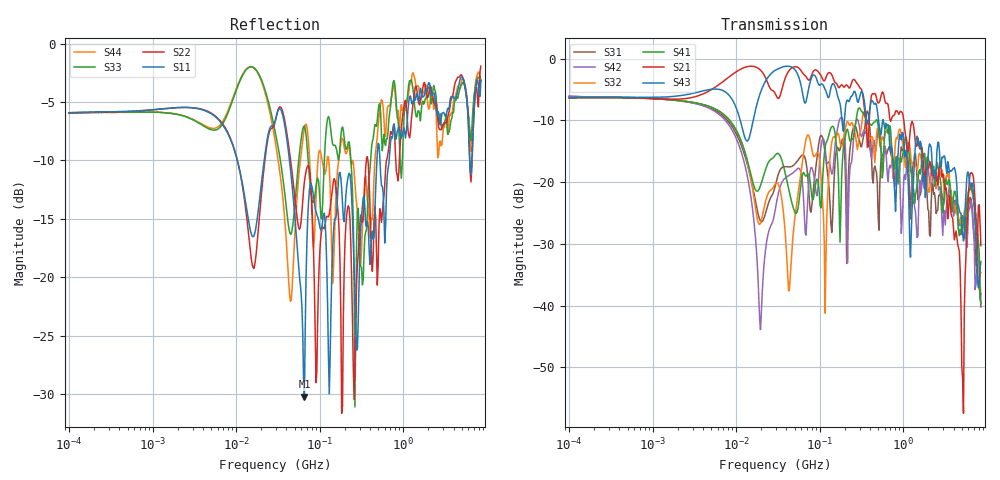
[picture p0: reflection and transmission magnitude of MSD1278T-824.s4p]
# MHz S MA R 50
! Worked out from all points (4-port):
!   498 points, 100 kHz to 8.5 GHz, reference 50 ohm
!   strongest paths, dB at 100 kHz, 1.698 MHz, 29.49 MHz, 500.7 MHz, 8.5 GHz:
!     S43: -6.3, -6.2, -1.9, -9.5, -32.8
!     S21: -6.4, -6.6, -5.7, -7.2, -30.3
!     S41: -6.4, -6.7, -15.6, -10.9, -39.5
!     S32: -6.4, -6.7, -20.3, -11.3, -34.7
!     S42: -6.1, -6.7, -24.4, -11.4, -38.0
!     S31: -6.1, -6.7, -20.5, -25.5, -40.2
!   lowest |S11| = -30.2 dB at 65.59 MHz (marker M1), VSWR 1.06, Z = 53.1 + j0.452 ohm
!   |S11| at or under -10 dB: 43.46 MHz to 484.3 MHz (440.9 MHz wide, 167 % of centre); 526.4 MHz to 678.1 MHz (151.7 MHz wide, 25.2 % of centre); 6.252 GHz to 6.618 GHz (365.6 MHz wide, 5.68 % of centre)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
0.1  0.5059 5.4  0.4812 6.1  0.4951 -7.2  0.4807 -175.5
     0.4812 6.1  0.5047 5.5  0.4805 -175.5  0.4953 -7.3
     0.4951 -7.2  0.4805 -175.5  0.5051 5.5  0.4826 6.0
     0.4807 -175.5  0.4953 -7.3  0.4826 6.0  0.5036 5.6
19.54962  0.2337 17.6  0.8058 -13.1  0.04836 -163.0  0.09366 69.0
          0.8058 -13.1  0.2051 29.1  0.04652 57.7  0.006398 29.0
          0.04836 -163.0  0.04652 57.7  0.7153 -33.3  0.5315 38.2
          0.09366 69.0  0.006398 29.0  0.5315 38.2  0.7061 -40.8
42.49738  0.3387 -68.9  0.7908 6.8  0.1325 92.8  0.08804 2.7
          0.7908 6.8  0.3657 -54.3  0.01314 43.2  0.1123 98.1
          0.1325 92.8  0.01314 43.2  0.1639 -37.2  0.8664 -8.5
          0.08804 2.7  0.1123 98.1  0.8664 -8.5  0.09594 -52.3
65.58595  0.03077 7.9  0.7368 -17.4  0.1619 6.4  0.1167 34.1
          0.7368 -17.4  0.2561 -25.7  0.1887 89.4  0.05253 17.7
          0.1619 6.4  0.1887 89.4  0.4425 -19.0  0.4435 -25.3
          0.1167 34.1  0.05253 17.7  0.4435 -25.3  0.434 -4.2
2840.13  0.4739 114.0  0.1251 -31.5  0.08799 80.3  0.09286 44.6
         0.1251 -31.5  0.4287 114.3  0.1129 74.3  0.06558 29.6
         0.08799 80.3  0.1129 74.3  0.4505 87.8  0.1338 76.9
         0.09286 44.6  0.06558 29.6  0.1338 76.9  0.3647 100.9
5142.985  0.7165 -103.1  0.002548 64.9  0.04315 -134.7  0.05339 -125.0
          0.002548 64.9  0.716 -104.7  0.04331 -118.8  0.05338 -150.2
          0.04315 -134.7  0.04331 -118.8  0.6804 -99.0  0.03843 112.7
          0.05339 -125.0  0.05338 -150.2  0.03843 112.7  0.7081 -97.7
8500  0.6942 -38.6  0.03058 -147.1  0.009782 -93.4  0.01053 -116.7
      0.03058 -147.1  0.8005 -43.9  0.01846 -100.8  0.01253 -77.6
      0.009782 -93.4  0.01846 -100.8  0.6916 -53.5  0.0228 -15.5
      0.01053 -116.7  0.01253 -77.6  0.0228 -15.5  0.6901 -54.9
